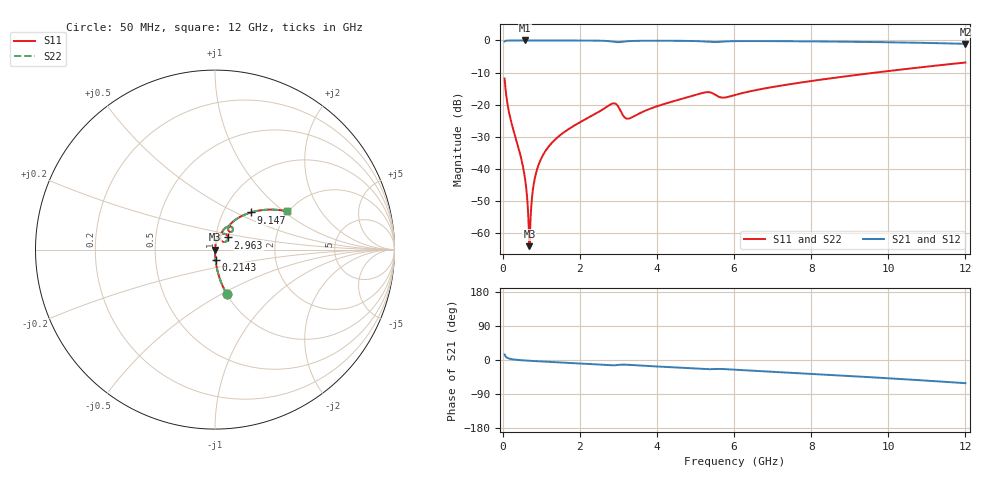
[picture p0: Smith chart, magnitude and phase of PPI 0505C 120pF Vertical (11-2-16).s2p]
# GHz S MA R 50
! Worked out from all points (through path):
!   1601 points, 50 MHz to 12 GHz, reference 50 ohm
!   highest |S21| = -0.01 dB at 580.3 MHz (marker M1); lowest = -1.1 dB at 12 GHz (marker M2)
!   group delay of S21, straight-line fit = 14.1 ps
!   lowest |S11| = -64.1 dB at 692.3 MHz (marker M3), VSWR 1.00, Z = 50.1 - j0.0141 ohm
!   |S11| at or under -10 dB: start of sweep to 9.684 GHz
!   |S22| runs from -64.1 to -6.9 dB; largest |S21 - S12| = 0
!   S11 on the Smith chart (normalised r, x): 50 MHz: 1.00, -0.53; 214.3 MHz: 1.00, -0.11; 2.963 GHz: 1.15, +0.16; 9.147 GHz: 1.34, +0.61; 12 GHz: 1.95, +1.05
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0.05  0.2547 -75.3  0.9668 14.6  0.9668 14.6  0.2547 -75.3
0.2143125  0.05582 -87.0  0.998 2.6  0.998 2.6  0.05582 -87.0
0.4757188  0.01482 -88.5  0.9993 -0.6  0.9993 -0.6  0.01482 -88.5
0.5802812  0.006942 -86.6  0.9994 -1.3  0.9994 -1.3  0.006942 -86.6
0.6549687  0.002326 -77.0  0.9994 -1.8  0.9994 -1.8  0.002326 -77.0
0.6923125  0.0006207 -13.1  0.9993 -2.0  0.9993 -2.0  0.0006207 -13.1
0.7296563  0.002 69.6  0.9993 -2.3  0.9993 -2.3  0.002 69.6
0.7894062  0.004987 80.0  0.9993 -2.6  0.9993 -2.6  0.004987 80.0
0.8491562  0.007834 82.2  0.9992 -2.9  0.9992 -2.9  0.007834 82.2
1.043344  0.01625 83.4  0.9991 -4.0  0.9991 -4.0  0.01625 83.4
1.416781  0.03063 82.4  0.9985 -5.9  0.9985 -5.9  0.03063 82.4
2.044156  0.05462 79.1  0.9967 -9.1  0.9967 -9.1  0.05462 79.1
2.813438  0.1018 60.4  0.9674 -13.9  0.9674 -13.9  0.1018 60.4
2.962813  0.09922 43.0  0.9415 -13.4  0.9415 -13.4  0.09922 43.0
3.246625  0.06021 51.9  0.9724 -12.6  0.9724 -12.6  0.06021 51.9
4.038312  0.09569 69.0  0.9889 -17.3  0.9889 -17.3  0.09569 69.0
5.255719  0.1551 55.9  0.9611 -24.1  0.9611 -24.1  0.1551 55.9
6.025  0.1409 58.4  0.9751 -25.6  0.9751 -25.6  0.1409 58.4
8.019156  0.2338 52.1  0.9669 -36.7  0.9669 -36.7  0.2338 52.1
9.146937  0.2883 45.9  0.9522 -43.1  0.9522 -43.1  0.2883 45.9
10.01331  0.3341 40.9  0.937 -48.3  0.937 -48.3  0.3341 40.9
12  0.4529 28.2  0.8853 -61.1  0.8853 -61.1  0.4529 28.2
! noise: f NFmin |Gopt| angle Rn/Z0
0.05  0.000345  0.8485  0.3515  0.0004844
1.372  0.003526  0.6393  3.864  0.001843
2.701  0.01977  0.8567  7.861  0.02935
4.031  0.01597  0.7513  11.57  0.01282
5.36  0.04594  0.8772  15.55  0.07939
6.682  0.0219  0.7092  18.81  0.01443
8.012  0.02035  0.6423  21.79  0.01039
9.341  0.02186  0.6205  24.79  0.01028
10.67  0.02432  0.6158  27.76  0.01114
12  0.02747  0.6214  30.73  0.01265
